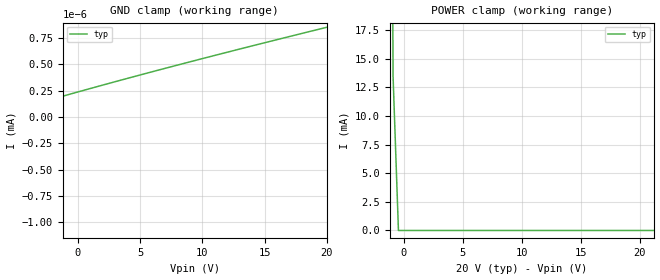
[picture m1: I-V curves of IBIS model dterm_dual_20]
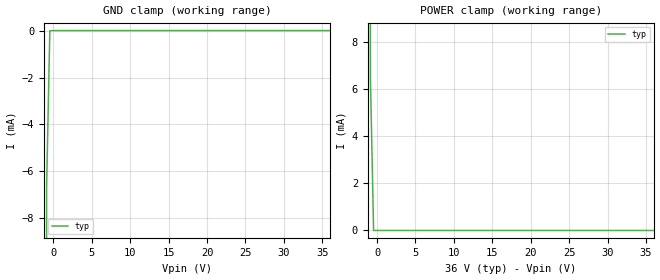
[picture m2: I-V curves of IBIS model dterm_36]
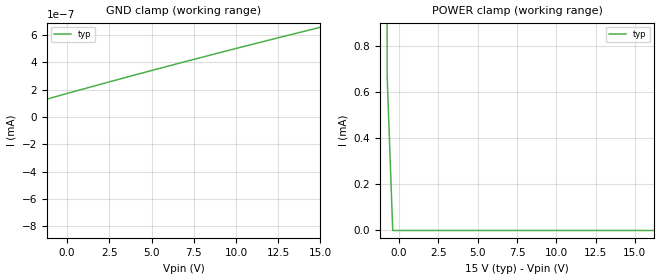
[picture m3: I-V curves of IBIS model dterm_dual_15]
|Texas Instruments Incorporated
|tmux7411f, 4 Channel 1:1 fault protected mux
[IBIS Ver]   4.1
[File name]   tmux7411f.ibs
[Date]   10/01/21
[File Rev]   1.0
[Source]
| Texas Instruments Incorporated.
| ASC-INT-MPD
| 12500 TI Blvd
| Dallas, TX - 75243
[Notes]   Revision History:
| Rev 1.0: 10/01/21
| - Initial version of the model
| - Model generated from simulations in SPECTRE
| - C_comp although listed in numerical order of value are
|   obtained from varying PVT conditions. For PVT conditions for
|   each specific value refer the buffer description under
|   respective [Model]. IBIS model user is responsible for using
|   appropriate C_comp to simulate for Signal Integrity.
[Disclaimer]
| This model is designed as an aid for customers of Texas Instruments.
| TI and its licensors and suppliers make no warranties, either expressed
| or implied, with respect to this  model, including the warranties of
| merchantability or fitness for a particular purpose. The model is
| provided solely on an "as is" basis. The entire risk as to its quality
| and performance is with the customer.
| This model is subject to change without notice. Texas Instruments
| Incorporated is not responsible for updating this model.
[Copyright]
(C) Copyright 2021 Texas Instruments Incorporated.All rights reserved.
|  Component TMUX7411FPW 16-pin - PW package
|  Part # TMUX7411FPW
[Component]   TMUX7411FPW
[Manufacturer]  TI
[Package]
|   typ   min   max
R_pkg   0.0668   NA   NA
L_pkg   2.1992nH   NA   NA
C_pkg   0.2884pF   NA   NA
[Pin]   signal_name   model_name
   1   SEL1   inbuf
   2   D1   dterm
   3   S1   sterm
   4   VSS   POWER
   5   GND   GND
   6   S4   sterm
   7   D4   dterm
   8   SEL4   inbuf
   9   SEL3   inbuf
   10   D3   dterm
   11   S3   sterm
   12   FF   NC
   13   VDD   POWER
   14   S2   sterm
   15   D2   dterm
   16   SEL2   inbuf
[Series Switch Groups]
On 1 /
On 2 /
On 3 /
On 4 /
Off 1 2 3 4 /
[Series Pin Mapping]  pin_2 model_name function_table_group
   3   2   switch_dual_20   1
  14  15   switch_dual_20   2
  11  10   switch_dual_20   3
   6   7   switch_dual_20   4
|   3   2   switch_36   1
|  14  15   switch_36   2
|  11  10   switch_36   3
|   6   7   switch_36   4
|   3   2   switch_dual_15   1
|  14  15   switch_dual_15   2
|  11  10   switch_dual_15   3
|   6   7   switch_dual_15   4
|   3   2   switch_12   1
|  14  15   switch_12   2
|  11  10   switch_12   3
|   6   7   switch_12   4
|  Component TMUX7411FRRQ 16-pin - RRQ package
|  Part # TMUX7411FRRQ
[Component]   TMUX7411FRRP
[Manufacturer]  TI
[Package]
|   typ   min   max
R_pkg   0.1   NA   NA
L_pkg   1.0nH   NA   NA
C_pkg   0.2pF   NA   NA
[Pin]   signal_name   model_name
   1   S1   sterm
   2   VSS   POWER
   3   GND   GND
   4   S4   sterm
   5   D4   dterm
   6   SEL4   inbuf
   7   SEL3   inbuf
   8   D3   dterm
   9   S3   sterm
   10   FF   NC
   11   VDD   POWER
   12   S2   sterm
   13   D2   dterm
   14   SEL2   inbuf
   15   SEL1   inbuf
   16   D1   dterm
[Series Switch Groups]
On 1 /
On 2 /
On 3 /
On 4 /
Off 1 2 3 4 /
[Series Pin Mapping]  pin_2 model_name function_table_group
   1  16   switch_dual_20   1
  12  13   switch_dual_20   2
   9   8   switch_dual_20   3
   5   4   switch_dual_20   4
|   1  16   switch_36   1
|  12  13   switch_36   2
|   9   8   switch_36   3
|   5   4   switch_36   4
|   1  16   switch_dual_15   1
|  12  13   switch_dual_15   2
|   9   8   switch_dual_15   3
|   5   4   switch_dual_15   4
|   1  16   switch_12   1
|  12  13   switch_12   2
|   9   8   switch_12   3
|   5   4   switch_12   4
[Model Selector] dterm
dterm_dual_20 Use for operation at +/-20V
dterm_36 Use for operation at 36V
dterm_dual_15 Use for operation at +/-15V
dterm_12 Use for operation at 12V
[Model Selector] sterm
sterm_dual_20 Use for operation at +/-20V
sterm_36 Use for operation at 36V
sterm_dual_15 Use for operation at +/-15V
sterm_12 Use for operation at 12V
[Model Selector] inbuf
inbuf_dual_20 Use for operation at +/-20V
inbuf_36 Use for operation at 36V
inbuf_dual_15 Use for operation at +/-15V
inbuf_12 Use for operation at 12V
| switch_dual_20
[Model]   switch_dual_20
Model_type   Series_switch
|   typ   min   max
C_comp   4.014581e-12   NA   NA
[Voltage Range]   20   NA   NA
[Power Clamp Reference]   20   NA   NA
[Temperature Range]   27   NA   NA
[On]
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[Off]
|   typ   min   max
[R Series]   10G   NA   NA
| switch_36
[Model]   switch_36
Model_type   Series_switch
|   typ   min   max
C_comp   4.014581e-12   NA   NA
[Voltage Range]   36   NA   NA
[Power Clamp Reference]   36   NA   NA
[Temperature Range]   27   NA   NA
[On]
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[Off]
|   typ   min   max
[R Series]   10G   NA   NA
| switch_dual_15
[Model]   switch_dual_15
Model_type   Series_switch
|   typ   min   max
C_comp   4.014581e-12   NA   NA
[Voltage Range]   15   NA   NA
[Power Clamp Reference]   15   NA   NA
[Temperature Range]   27   NA   NA
[On]
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[Off]
|   typ   min   max
[R Series]   10G   NA   NA
| switch_12
[Model]   switch_12
Model_type   Series_switch
|   typ   min   max
C_comp   6.362683e-12   NA   NA
[Voltage Range]   12   NA   NA
[Power Clamp Reference]   12   NA   NA
[Temperature Range]   27   NA   NA
[On]
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[Off]
|   typ   min   max
[R Series]   10G   NA   NA
| Models and submodels in the file (16): dterm_dual_20 (Terminator), dterm_36 (Terminator), dterm_dual_15 (Terminator), dterm_12 (Terminator), switch_dual_20 (Series_switch), switch_36 (Series_switch), switch_dual_15 (Series_switch), switch_12 (Series_switch), sterm_dual_20 (Terminator), sterm_36 (Terminator), sterm_dual_15 (Terminator), sterm_12 (Terminator), inbuf_dual_20 (Input), inbuf_36 (Input), inbuf_dual_15 (Input), inbuf_12 (Input)
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| dterm_dual_20
[Model]   dterm_dual_20
Model_type   Terminator
|   typ   min   max
C_comp   4.014581e-12   NA   NA
[Voltage Range]   20   NA   NA
[Temperature Range]   27   NA   NA
[Power Clamp Reference]   20   NA   NA
[GND Clamp Reference]   0   NA   NA
[GND Clamp]
|   Voltage   I(typ)   I(min)   I(max)
-25V      -1.049A    NA         NA
-20.45V   -11.62uA   NA         NA
-20V      -718.2pA   NA         NA
-19.55V   -396.8pA   NA         NA
-14.09V   -242.2pA   NA         NA
-2.273V   162.5pA    NA         NA
5V        399.5pA    NA         NA
20V       853.1pA    NA         NA
[POWER Clamp]
|   Voltage   I(typ)   I(min)   I(max)
-5V       1.049A     NA         NA
-1.364V   115.2mA    NA         NA
-909.1mV  13.42mA    NA         NA
-454.5mV  62.28nA    NA         NA
40V       -718.2pA   NA         NA
| dterm_36
[Model]   dterm_36
Model_type   Terminator
|   typ   min   max
C_comp   4.014581e-12   NA   NA
[Voltage Range]   36   NA   NA
[Temperature Range]   27   NA   NA
[Power Clamp Reference]   36   NA   NA
[GND Clamp Reference]   0   NA   NA
[GND Clamp]
|   Voltage   I(typ)   I(min)   I(max)
-5V       -1.049A    NA         NA
-1.273V   -93.04mA   NA         NA
-858.6mV  -6.554mA   NA         NA
-444.4mV  -8.49uA    NA         NA
36V       776.4pA    NA         NA
[POWER Clamp]
|   Voltage   I(typ)   I(min)   I(max)
-5V       1.049A     NA         NA
-1.273V   93.03mA    NA         NA
-858.6mV  6.542mA    NA         NA
-444.4mV  45.69nA    NA         NA
36V       -563.9pA   NA         NA
| dterm_dual_15
[Model]   dterm_dual_15
Model_type   Terminator
|   typ   min   max
C_comp   4.014581e-12   NA   NA
[Voltage Range]   15   NA   NA
[Temperature Range]   27   NA   NA
[Power Clamp Reference]   15   NA   NA
[GND Clamp Reference]   0   NA   NA
[GND Clamp]
|   Voltage   I(typ)   I(min)   I(max)
-20V      -1.049A    NA         NA
-15.05V   -2.336nA   NA         NA
-14.7V    -297pA     NA         NA
-11.52V   -212.6pA   NA         NA
-9.04V    -137.2pA   NA         NA
4.394V    320.6pA    NA         NA
15V       657pA      NA         NA
[POWER Clamp]
|   Voltage   I(typ)   I(min)   I(max)
-5V       1.049A     NA         NA
-1.111V   54.85mA    NA         NA
-757.6mV  668.1uA    NA         NA
-404mV    12.71nA    NA         NA
30V       -599.2pA   NA         NA
